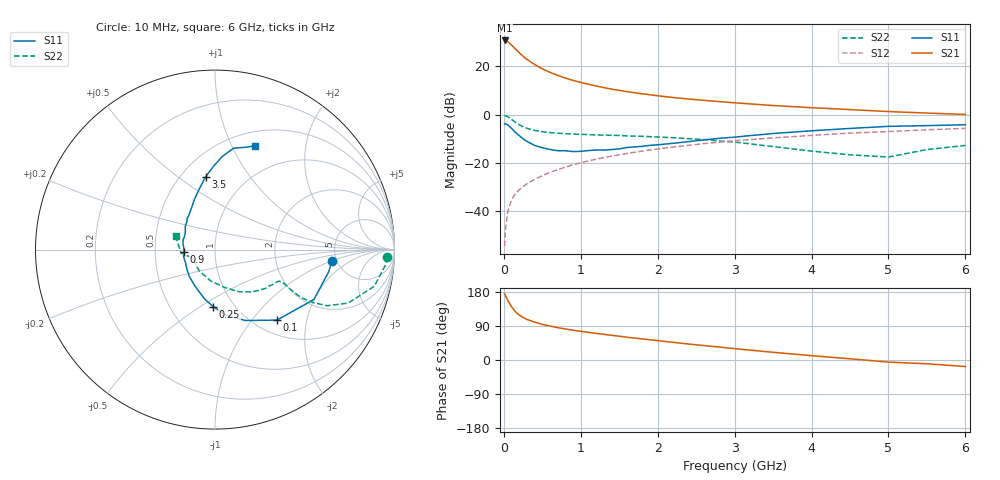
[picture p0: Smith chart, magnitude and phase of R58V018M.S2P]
! SIEMENS Small Signal Semiconductors
! BFR183
! Si NPN RF Bipolar Junction Transistor in SOT23
! VCE = 8 V  IC = 18 mA
! Common Emitter S-Parameters:  May  1996
# GHz  S  MA  R  50
!  f  S11  S21  S12  S22
! GHz  MAG  ANG  MAG  ANG  MAG  ANG  MAG  ANG
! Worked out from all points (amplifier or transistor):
!   36 points, 10 MHz to 6 GHz, reference 50 ohm
!   highest |S21| = 30.7 dB at 10 MHz (marker M1)
!   |S21| within 3 dB of that: start of sweep to 133.8 MHz
!   unconditionally stable (mu >= 1): 652.6 MHz to 2.533 GHz
!   at 250 MHz: K = 0.75, MSG = 26.9 dB, |S12| = -29.7 dB
!   at 1.4 GHz: K = 1.05, MAG = 12.6 dB, |S12| = -17.2 dB
!   at 6 GHz: K = 0.90, MSG = 2.9 dB, |S12| = -5.7 dB
!   S11 on the Smith chart (normalised r, x): 10 MHz: 4.53, -1.01; 100 MHz: 1.25, -1.35; 250 MHz: 0.80, -0.57; 900 MHz: 0.71, -0.02; 3.5 GHz: 0.65, +0.64; 6 GHz: 0.66, +1.24
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0.01  0.6533 -5.6  34.44 174.7  0.0019 90.1  0.9615 -2.5
0.02  0.6461 -10.9  34.06 170.2  0.004 82.9  0.953 -5.3
0.05  0.617 -26.8  32.57 157.8  0.0098 79.7  0.9104 -13.0
0.1  0.5229 -48.7  27.68 140.6  0.0174 71.1  0.7989 -21.9
0.15  0.4294 -66.9  22.94 127.4  0.0231 67.9  0.6982 -26.6
0.2  0.3697 -80.6  19.18 118.6  0.028 68.0  0.6194 -28.4
0.25  0.3177 -91.8  16.2 112.2  0.0327 67.2  0.5627 -29.0
0.3  0.2808 -102.0  13.99 107.0  0.0372 68.0  0.5248 -28.8
0.4  0.2311 -119.1  10.96 99.9  0.0458 68.6  0.4735 -27.7
0.5  0.2072 -133.6  8.894 94.0  0.0547 69.4  0.4436 -26.7
0.6  0.1905 -145.2  7.53 89.5  0.0641 69.6  0.4267 -26.1
0.7  0.1801 -155.4  6.525 85.4  0.0729 70.1  0.4145 -26.1
0.9  0.1726 -174.9  5.13 78.6  0.0921 69.4  0.3969 -26.3
1.1  0.1813 169.3  4.269 73.0  0.1106 68.4  0.3874 -28.1
1.3  0.1848 157.6  3.638 67.7  0.1295 66.8  0.3785 -29.9
1.6  0.2094 142.5  3 60.1  0.1575 64.2  0.3646 -33.6
2.2  0.2558 122.3  2.27 46.6  0.2142 58.3  0.3348 -43.0
3.5  0.4089 97.4  1.549 20.3  0.3311 42.3  0.2191 -75.2
4.5  0.5201 85.6  1.276 3.2  0.4164 30.2  0.1479 -126.9
5  0.5742 79.6  1.162 -5.5  0.4478 22.9  0.133 -159.5
5.5  0.5943 73.6  1.082 -10.0  0.4869 18.8  0.1899 -174.3
6  0.6201 68.7  1.013 -17.2  0.5212 11.4  0.2312 161.3
